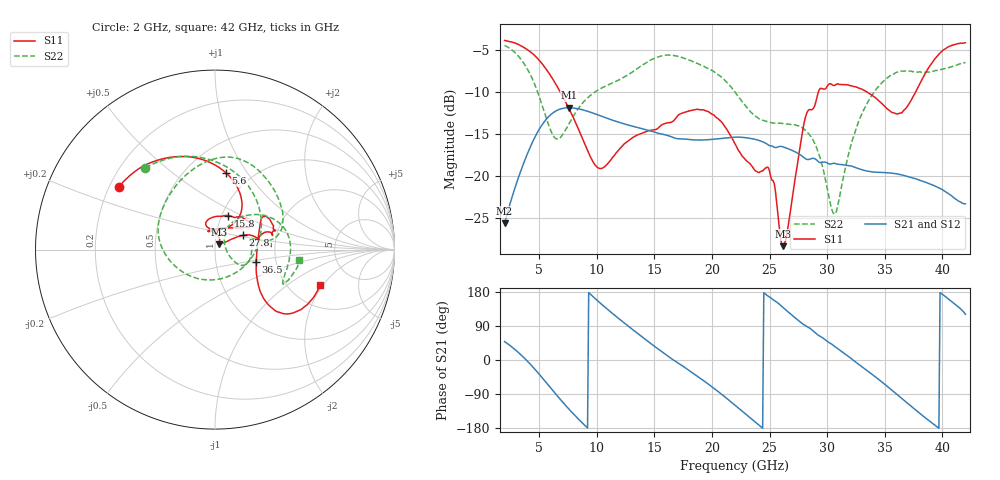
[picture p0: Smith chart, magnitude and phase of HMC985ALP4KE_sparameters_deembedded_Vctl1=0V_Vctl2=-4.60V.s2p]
!s2p File: Measurements: S11, S21, S12, S22
# GHz S dB R 50.0
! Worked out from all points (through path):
!   401 points, 2 GHz to 42 GHz, reference 50 ohm
!   highest |S21| = -11.89 dB at 7.6 GHz (marker M1); lowest = -25.7 dB at 2 GHz (marker M2)
!   lowest |S11| = -28.4 dB at 26.2 GHz (marker M3), VSWR 1.08, Z = 52.3 + j3.18 ohm
!   |S11| at or under -10 dB: 6.82 GHz to 29.25 GHz (22.43 GHz wide, 124 % of centre); 33.42 GHz to 37.69 GHz (4.267 GHz wide, 12 % of centre)
!   |S22| runs from -24.6 to -4.5 dB; largest |S21 - S12| = 0.00024
!   S11 on the Smith chart (normalised r, x): 2 GHz: 0.24, +0.28; 5.6 GHz: 0.76, +0.80; 15.8 GHz: 1.07, +0.42; 27.8 GHz: 1.34, +0.22; 36.5 GHz: 1.57, -0.23; 42 GHz: 2.94, -1.89
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2  -3.88 147.0  -25.66 48.6  -25.67 48.6  -4.47 130.5
3.6  -4.66 120.3  -18.70 8.4  -18.70 8.4  -6.47 84.9
4.7  -5.80 99.5  -15.21 -26.8  -15.22 -26.8  -9.41 43.4
5.6  -7.29 81.9  -13.29 -59.0  -13.30 -59.0  -13.04 -3.7
6.5  -9.22 66.5  -12.24 -92.0  -12.25 -92.0  -15.60 -68.9
7.6  -12.04 54.8  -11.89 -130.1  -11.90 -130.1  -13.77 -135.7
8.7  -15.38 55.1  -12.12 -164.7  -12.12 -164.7  -11.45 -170.2
10.4  -19.13 89.6  -12.90 147.6  -12.90 147.5  -9.57 162.5
15.4  -14.23 75.7  -14.97 27.6  -14.97 27.5  -5.80 87.2
15.8  -13.83 68.7  -15.07 18.6  -15.07 18.6  -5.67 82.1
19.4  -12.23 33.3  -15.72 -57.2  -15.72 -57.2  -7.04 35.1
22  -16.18 51.1  -15.40 -119.3  -15.41 -119.3  -10.03 9.9
24.9  -19.04 104.8  -16.34 168.0  -16.34 168.0  -13.59 13.2
26.2  -28.38 52.8  -16.57 137.6  -16.58 137.5  -13.79 -2.4
27.8  -15.23 27.2  -17.64 97.1  -17.64 97.0  -14.24 -24.3
28.7  -12.11 12.6  -17.93 78.9  -17.93 78.9  -15.55 -31.3
30.7  -9.21 20.7  -18.53 34.7  -18.53 34.6  -24.53 22.3
32.8  -9.59 33.9  -19.18 -12.9  -19.19 -13.0  -13.29 53.5
35.4  -12.22 11.8  -19.66 -74.1  -19.66 -74.2  -8.17 21.6
36.5  -12.47 -16.7  -19.90 -102.0  -19.91 -102.0  -7.53 7.5
39.5  -5.85 -43.8  -21.31 -175.3  -21.30 -175.4  -7.45 -26.3
42  -4.16 -18.6  -23.33 120.5  -23.34 120.5  -6.48 -7.2
